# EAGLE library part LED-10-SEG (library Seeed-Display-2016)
304080004
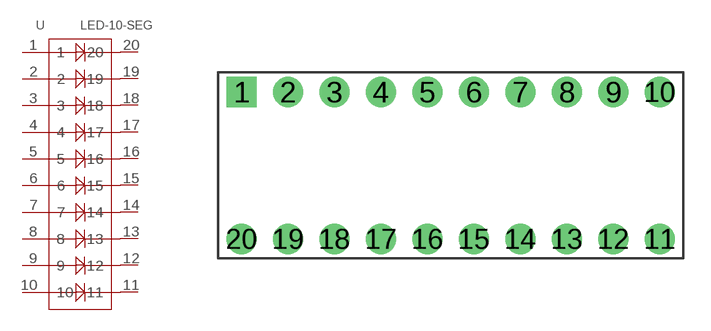
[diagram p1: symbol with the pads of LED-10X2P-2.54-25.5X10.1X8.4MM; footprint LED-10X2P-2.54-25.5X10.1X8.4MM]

Designator prefix U

## LED-10-SEG'SB1K1Y8G'  [LED-10X2P-2.54-25.5X10.1X8.4MM]
1  1
2  2
3  3
4  4
5  5
6  6
7  7
8  8
9  9
10  10
11  11
12  12
13  13
14  14
15  15
16  16
17  17
18  18
19  19
20  20

## Footprint LED-10X2P-2.54-25.5X10.1X8.4MM (pad centres in mm)
drill 0.889 pad 1.651 square: 1 -11.43,4.013
drill 0.889 pad 1.651: 2 -8.89,4.013; 3 -6.35,4.013; 4 -3.81,4.013; 5 -1.27,4.013; 6 1.27,4.013; 7 3.81,4.013; 8 6.35,4.013; 9 8.89,4.013; 10 11.43,4.013; 11 11.43,-4.013; 12 8.89,-4.013; 13 6.35,-4.013; 14 3.81,-4.013; 15 1.27,-4.013; 16 -1.27,-4.013; 17 -3.81,-4.013; 18 -6.35,-4.013; 19 -8.89,-4.013; 20 -11.43,-4.013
